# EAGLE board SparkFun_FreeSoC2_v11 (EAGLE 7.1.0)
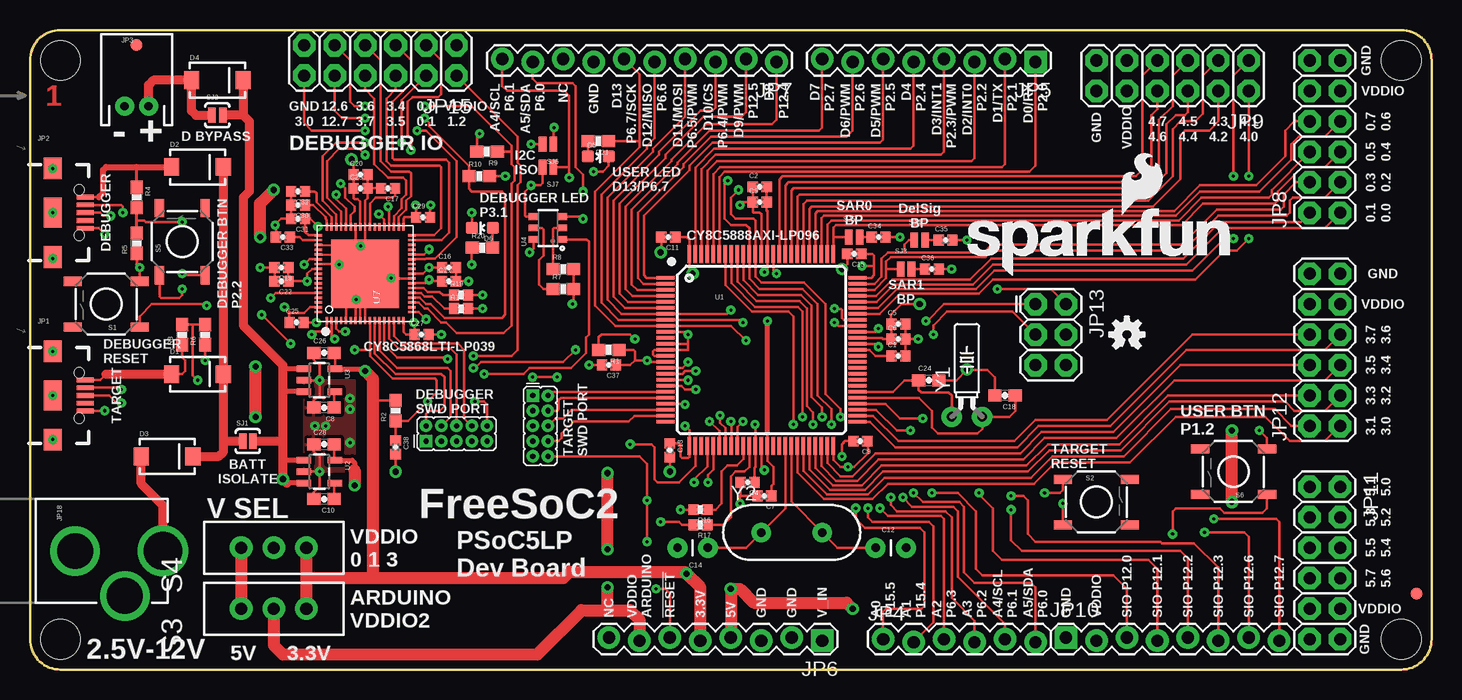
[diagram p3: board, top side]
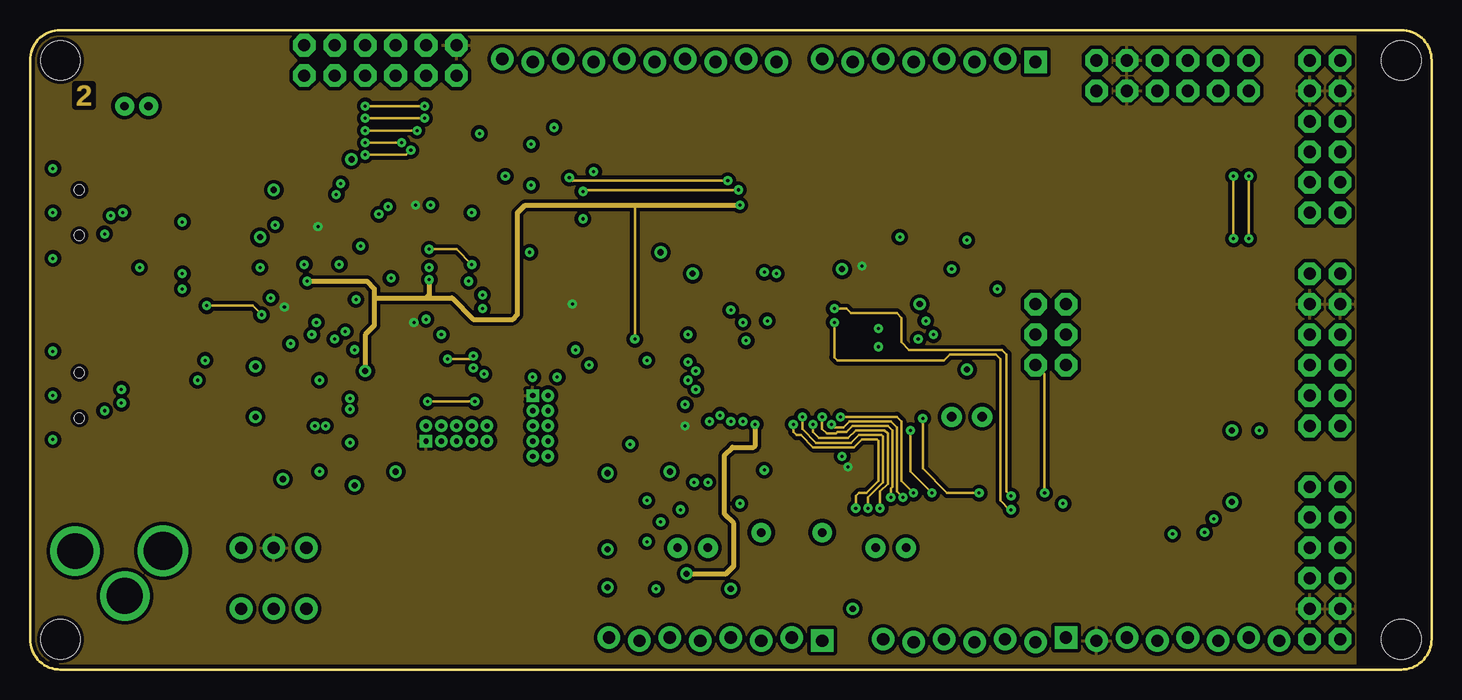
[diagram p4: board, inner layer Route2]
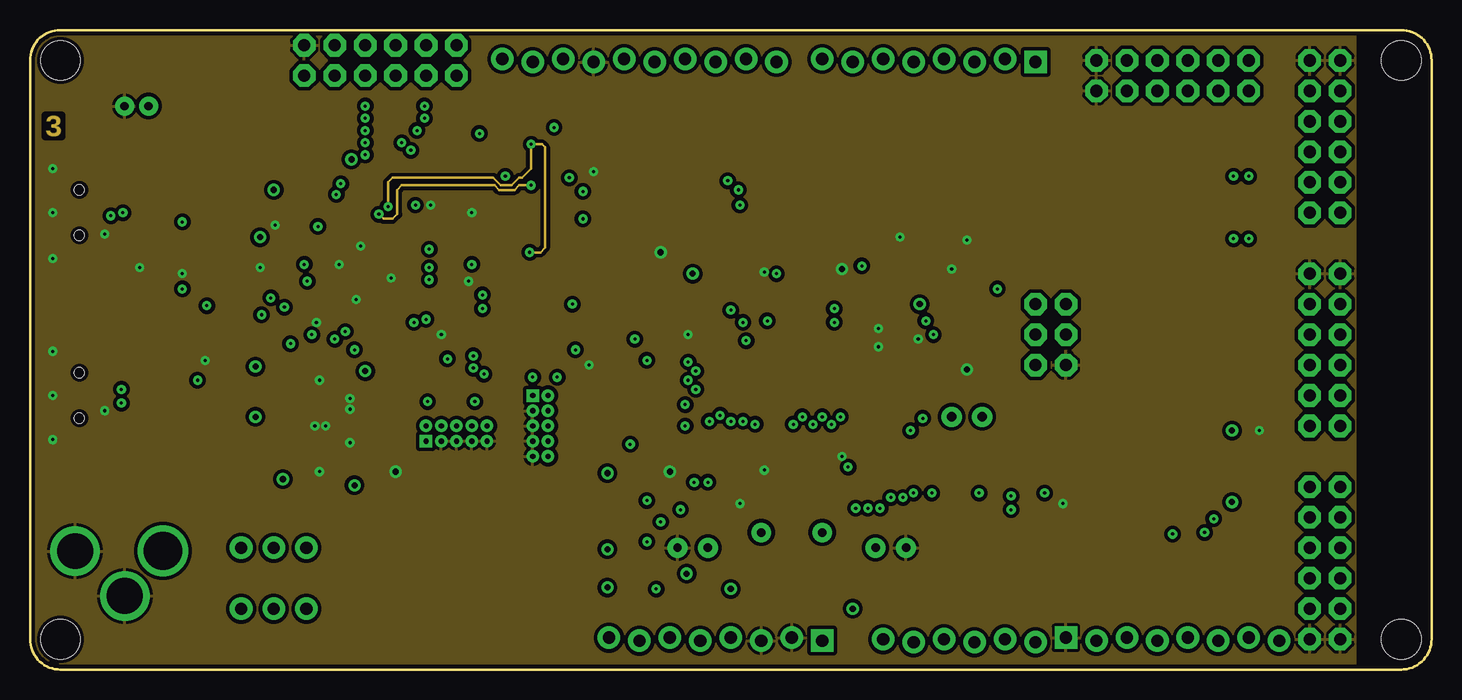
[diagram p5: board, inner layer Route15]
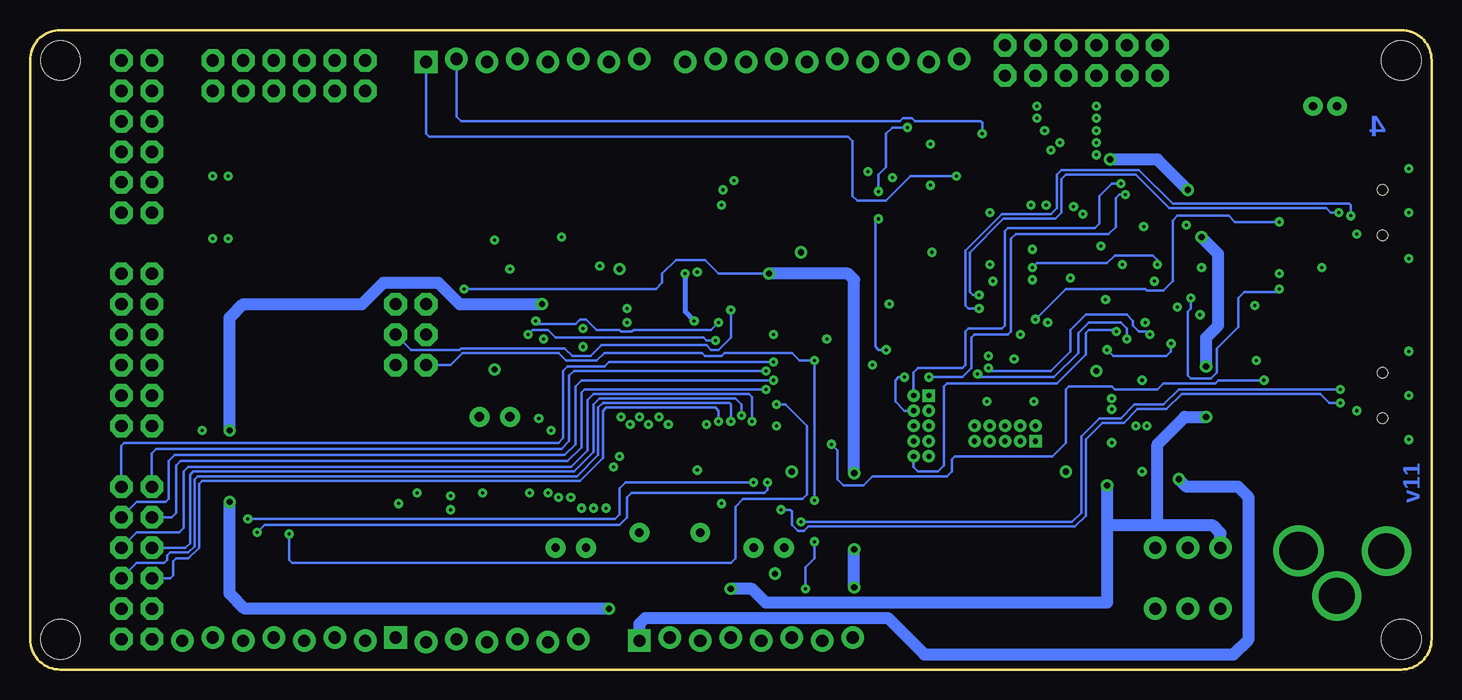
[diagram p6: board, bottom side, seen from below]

Size 116.84 x 53.34 mm. Coordinates in mm from the lower left corner, seen from the top.
Outline: 114.3,0 2.54,0 arc-90 0,2.54 0,50.8 arc-90 2.54,53.34 114.3,53.34 arc-90 116.84,50.8 116.84,2.54 arc-90 114.3,0
Copper layers (1*2*15*16): Top 0.035mm / dielectric 1.5mm / Route2 0.035mm / dielectric 0.15mm / Route15 0.035mm / dielectric 0.2mm / Bottom 0.035mm
Design rules "Sparkfun-x *": minimum track width 6mil, minimum drill 10mil, track to track 6mil, track to pad 6mil, pad to pad 6mil, via to via 8mil, smd to smd 6mil, copper to edge 6mil, drill to drill 8mil, minimum pad ring 12mil, minimum via ring 10mil, stop-mask expansion 4mil, vias tented up to drill 20mil, thermal gap 10mil
Net classes: 0 signal: width 0.203 mm, drill 0.254 mm, clearance 0.152 mm; 1 AVCC: width 0.508 mm, drill 0.508 mm, clearance 0.152 mm; 2 ARDUINO_VCC: width 0.508 mm, drill 0.381 mm

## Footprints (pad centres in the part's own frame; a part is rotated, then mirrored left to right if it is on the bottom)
0402-CAP = smd 0.85 x 0.9: 1 -0.58,0; 2 0.58,0
0603-CAP = smd 1.1 x 1: 1 -0.85,0; 2 0.85,0
CAP-PTH-SMALL = drill 0.7 pad 1.651: 1 0,0; 2 2.54,0
SMA-DIODE = smd 1.27 x 1.47: A -2.15,0; C 2.15,0
LED-0603 = smd 1 x 1: A 0,-0.877; C 0,0.877
FIDUCIAL-1X2 = smd 1 x 1: 1 0,0
USB-B-MICRO-SMD_V03 = smd 1.4 x 0.4: D+1 2.7,0; D-1 2.7,0.65; GND1 2.7,-1.3; ID1 2.7,-0.65; VBUS1 2.7,1.3 | smd 1.5 x 1.8: SHIELD1 0,3.7; SHIELD2 0,-3.7 | smd 1.5 x 2.5: SHIELD3 0,0 | hole 0.85: 2.2,1.9; 2.2,-1.9
JST-2-PTH = drill 0.7 pad 1.6: 1 -1,0; 2 1,0
1X06-SIP_LOCK = drill 1.016 pad 1.88: 1 0,0; 2 2.54,-0.254; 3 5.08,0; 4 7.62,-0.254; 5 10.16,0; 6 12.7,-0.254
1X08_LOCK = drill 1.016 pad 1.88 square: 1 0,0.127 | drill 1.016 pad 1.88: 2 2.54,-0.127; 3 5.08,0.127; 4 7.62,-0.127; 5 10.16,0.127; 6 12.7,-0.127; 7 15.24,0.127; 8 17.78,-0.127
1X10_LOCK = drill 1.016 pad 1.88: 1 0,0.127; 2 2.54,-0.127; 3 5.08,0.127; 4 7.62,-0.127; 5 10.16,0.127; 6 12.7,-0.127; 7 15.24,0.127; 8 17.78,-0.127; 9 20.32,0.127; 10 22.86,-0.127
2X6 = drill 1.016 pad 1.88 octagon: 1 0,0; 2 0,2.54; 3 2.54,0; 4 2.54,2.54; 5 5.08,0; 6 5.08,2.54; 7 7.62,0; 8 7.62,2.54; 9 10.16,0; 10 10.16,2.54; 11 12.7,0; 12 12.7,2.54
2X3 = drill 1.016 pad 1.88 octagon: 1 0,0; 2 0,2.54; 3 2.54,0; 4 2.54,2.54; 5 5.08,0; 6 5.08,2.54
2X5_PTH_SILK_.05 = drill 0.432 square: 1 0,6.35 | drill 0.432: 2 1.27,6.35; 3 0,5.08; 4 1.27,5.08; 5 0,3.81; 6 1.27,3.81; 7 0,2.54; 8 1.27,2.54; 9 0,1.27; 10 1.27,1.27
POWER_JACK_PTH_LOCK = drill 2.997 pad 4.115: GND 0.025,6.557; GNDBREAK 3.762,10.7 | drill 3.2 pad 4.115: PWR 0,13.878
0603-RES = smd 1.1 x 1: 1 -0.85,0; 2 0.85,0
0402-RES = smd 0.85 x 0.9: 1 -0.58,0; 2 0.58,0
TACTILE-SWITCH-SMD = smd 1.524 x 0.762: 1 -2.794,1.905; 2 2.794,1.905; 3 -2.794,-1.905; 4 2.794,-1.905
SWITCH-SPDT_LOCK.007S = drill 1.016 pad 1.88: 1 0,2.718; 2 0,0; 3 0,-2.718
PAD-JUMPER-2-NC_BY_PASTE_YES_SILK = smd 0.635 x 1.27: 1 -0.401,0; 2 0.413,0
PAD-JUMPER-2-NO_YES_SILK = smd 0.635 x 1.27: 1 -0.45,0; 2 0.45,0
PAD-JUMPER-2-NO_NO_SILK = smd 0.635 x 1.27: 1 -0.45,0; 2 0.45,0
STAND-OFF = hole 3.302: 0,0
TQFP-100-14X14MM = smd 1.5 x 0.27: 1 -8,6; 2 -8,5.5; 3 -8,5; 4 -8,4.5; 5 -8,4; 6 -8,3.5; 7 -8,3; 8 -8,2.5; 9 -8,2; 10 -8,1.5; 11 -8,1; 12 -8,0.5; 13 -8,0; 14 -8,-0.5; 15 -8,-1; 16 -8,-1.5; 17 -8,-2; 18 -8,-2.5; 19 -8,-3; 20 -8,-3.5; 21 -8,-4; 22 -8,-4.5; 23 -8,-5; 24 -8,-5.5; 25 -8,-6; 51 8,-6; 52 8,-5.5; 53 8,-5; 54 8,-4.5; 55 8,-4; 56 8,-3.5; 57 8,-3; 58 8,-2.5; 59 8,-2; 60 8,-1.5; 61 8,-1; 62 8,-0.5; 63 8,0; 64 8,0.5; 65 8,1; 66 8,1.5; 67 8,2; 68 8,2.5; 69 8,3; 70 8,3.5; 71 8,4; 72 8,4.5; 73 8,5; 74 8,5.5; 75 8,6 | smd 0.27 x 1.5: 26 -6,-8; 27 -5.5,-8; 28 -5,-8; 29 -4.5,-8; 30 -4,-8; 31 -3.5,-8; 32 -3,-8; 33 -2.5,-8; 34 -2,-8; 35 -1.5,-8; 36 -1,-8; 37 -0.5,-8; 38 0,-8; 39 0.5,-8; 40 1,-8; 41 1.5,-8; 42 2,-8; 43 2.5,-8; 44 3,-8; 45 3.5,-8; 46 4,-8; 47 4.5,-8; 48 5,-8; 49 5.5,-8; 50 6,-8; 76 6,8; 77 5.5,8; 78 5,8; 79 4.5,8; 80 4,8; 81 3.5,8; 82 3,8; 83 2.5,8; 84 2,8; 85 1.5,8; 86 1,8; 87 0.5,8; 88 0,8; 89 -0.5,8; 90 -1,8; 91 -1.5,8; 92 -2,8; 93 -2.5,8; 94 -3,8; 95 -3.5,8; 96 -4,8; 97 -4.5,8; 98 -5,8; 99 -5.5,8; 100 -6,8
SOT23-5 = smd 0.55 x 1.2: 1 -0.95,-1.3; 2 0,-1.3; 3 0.95,-1.3; 4 0.95,1.3; 5 -0.95,1.3
SOT26 = smd 0.55 x 0.8: D1 -0.95,1.2; D2 0.95,1.2; G1 -0.95,-1.2; G2 0.95,-1.2; S1 0,1.2; S2 0,-1.2
QFN-68 = smd 0.6 x 0.2: 1 -3.9,3.2; 2 -3.9,2.8; 3 -3.9,2.4; 4 -3.9,2; 5 -3.9,1.6; 6 -3.9,1.2; 7 -3.9,0.8; 8 -3.9,0.4; 9 -3.9,0; 10 -3.9,-0.4; 11 -3.9,-0.8; 12 -3.9,-1.2; 13 -3.9,-1.6; 14 -3.9,-2; 15 -3.9,-2.4; 16 -3.9,-2.8; 17 -3.9,-3.2; 35 3.9,-3.2; 36 3.9,-2.8; 37 3.9,-2.4; 38 3.9,-2; 39 3.9,-1.6; 40 3.9,-1.2; 41 3.9,-0.8; 42 3.9,-0.4; 43 3.9,0; 44 3.9,0.4; 45 3.9,0.8; 46 3.9,1.2; 47 3.9,1.6; 48 3.9,2; 49 3.9,2.4; 50 3.9,2.8; 51 3.9,3.2 | smd 0.2 x 0.6: 18 -3.2,-3.9; 19 -2.8,-3.9; 20 -2.4,-3.9; 21 -2,-3.9; 22 -1.6,-3.9; 23 -1.2,-3.9; 24 -0.8,-3.9; 25 -0.4,-3.9; 26 0,-3.9; 27 0.4,-3.9; 28 0.8,-3.9; 29 1.2,-3.9; 30 1.6,-3.9; 31 2,-3.9; 32 2.4,-3.9; 33 2.8,-3.9; 34 3.2,-3.9; 52 3.2,3.9; 53 2.8,3.9; 54 2.4,3.9; 55 2,3.9; 56 1.6,3.9; 57 1.2,3.9; 58 0.8,3.9; 59 0.4,3.9; 60 0,3.9; 61 -0.4,3.9; 62 -0.8,3.9; 63 -1.2,3.9; 64 -1.6,3.9; 65 -2,3.9; 66 -2.4,3.9; 67 -2.8,3.9; 68 -3.2,3.9 | smd 5.7 x 5.7: 69 0,0
TC26H = drill 0.813 pad 1.676: 1 -1.27,0; 2 1.27,0
HC49US = drill 0.7 pad 1.651: 1 -2.54,0; 2 2.54,0

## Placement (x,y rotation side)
C1  1.0uF  [0402-CAP]  72.39,26.16 0 top
C2  1.0uF  [0402-CAP]  60.83,40.26 0 top
C3  0.1uF  [0402-CAP]  60.83,38.99 0 top
C4  1.0uF  [0402-CAP]  59.82,15.62 180 top
C5  1.0uF  [0402-CAP]  72.39,28.83 0 top
C6  0.1uF  [0402-CAP]  72.39,27.56 0 top
C7  1.0uF  [0402-CAP]  61.21,14.48 180 top
C8  470pF  [0603-CAP]  24.51,21.84 180 top
C9  0.1uF  [0402-CAP]  69.22,19.05 180 top
C10  470pF  [0603-CAP]  24.51,14.22 180 top
C11  0.1uF  [0402-CAP]  53.21,36.07 180 top
C12  [CAP-PTH-SMALL]  70.48,10.16 0 top
C13  0.1uF  [0402-CAP]  53.34,18.29 270 top
C14  [CAP-PTH-SMALL]  56.52,10.16 180 top
C15  0.1uF  [0402-CAP]  68.71,34.67 180 top
C16  1.0uF  [0402-CAP]  34.92,33.53 0 top
C17  1.0uF  [0402-CAP]  29.84,40.13 180 top
C18  22pF  [0603-CAP]  81.28,22.86 180 top
C19  1.0uF  [0402-CAP]  20.95,33.53 180 top
C20  1.0uF  [0402-CAP]  27.56,41.27 0 top
C21  0.1uF  [0402-CAP]  34.92,32.38 0 top
C22  0.1uF  [0402-CAP]  20.95,32.38 180 top
C23  0.1uF  [0402-CAP]  27.56,40.13 0 top
C24  22pF  [0603-CAP]  74.93,24.13 0 top
C25  0.1uF  [0402-CAP]  22.23,28.96 0 top
C26  2.2uF  [0603-CAP]  24.51,26.42 0 top
C27  0.1uF  [0402-CAP]  32.64,27.94 0 top
C28  2.2uF  [0603-CAP]  24.51,18.8 0 top
C29  0.1uF  [0402-CAP]  32.77,37.72 0 top
C30  0.1uF  [0402-CAP]  22.35,38.73 180 top
C31  0.1uF  [0402-CAP]  22.35,37.59 180 top
C32  0.1uF  [0402-CAP]  22.35,39.88 180 top
C33  0.1uF  [0402-CAP]  21.08,36.07 180 top
C34  0.1uF  [0402-CAP]  70.74,36.07 0 top
C35  0.1uF  [0402-CAP]  76.33,35.81 0 top
C36  0.1uF  [0402-CAP]  75.18,33.4 0 top
C37  0.1uF  [0402-CAP]  48.26,25.4 180 top
C38  0.1uF  [0402-CAP]  30.48,18.54 270 top
D1  MBRA140  [SMA-DIODE]  13.97,24.64 0 top
D2  MBRA140  [SMA-DIODE]  13.97,41.91 0 top
D3  MBRA140  [SMA-DIODE]  11.43,17.78 0 top
D4  MBRA140  [SMA-DIODE]  15.62,49.15 0 top
D5  RED  [LED-0603]  47.37,42.8 270 top
D6  RED  [LED-0603]  37.72,36.83 90 top
FID1  FIDUCIAL1X2  [FIDUCIAL-1X2]  115.57,6.35 0 top
FID2  FIDUCIAL1X2  [FIDUCIAL-1X2]  8.89,52.07 0 top
FRAME1  [DUMMY]  not placed on the board
FRAME2  [DUMMY]  not placed on the board
FRAME3  [DUMMY]  not placed on the board
JP1  MicroB  [USB-B-MICRO-SMD_V03]  1.91,22.86 0 top
JP2  MicroB  [USB-B-MICRO-SMD_V03]  1.91,38.1 0 top
JP3  M02JST-PTH-2  [JST-2-PTH]  8.89,46.99 0 top
JP4  1X6 FEMALE PTH  [1X06-SIP_LOCK]  71.12,2.54 0 top
JP5  1X8 FEMALE PTH  [1X08_LOCK]  83.82,50.8 180 top
JP6  1X8 FEMALE PTH  [1X08_LOCK]  66.04,2.54 180 top
JP7  1X10 FEMALE PTH  [1X10_LOCK]  62.23,50.8 180 top
JP8  2X6 FEMALE  [2X6]  109.22,38.1 90 top
JP9  2X6 FEMALE  [2X6]  101.6,50.8 180 top
JP10  1x8 FEMALE PTH  [1X08_LOCK]  86.36,2.54 0 top
JP11  2X6 FEMALE  [2X6]  106.68,15.24 270 top
JP12  2X6 FEMALE  [2X6]  109.22,20.32 90 top
JP13  [2X3]  83.82,30.48 270 top
JP14  DNP  [2X5_PTH_SILK_.05]  39.37,19.05 90 top
JP15  2X6 FEMALE  [2X6]  35.56,52.07 180 top
JP17  DNP  [2X5_PTH_SILK_.05]  41.91,16.51 0 top
JP18  POWER_JACKPTH_LOCK  [POWER_JACK_PTH_LOCK]  -2.79,9.91 270 top
LOGO1  SFE_LOGO_NAME_FLAME.2_INCH  [SFE_LOGO_NAME_FLAME_.2]  77.47,32.77 0 top
LOGO2  OSHW-LOGOS  [OSHW-LOGO-S]  91.44,27.94 0 top
R1  4.7K  [0603-RES]  48.26,26.67 180 top
R2  4.7K  [0603-RES]  30.48,21.59 90 top
R3  10K  [0603-RES]  12.7,27.94 90 top
R4  10K  [0603-RES]  8.89,39.37 270 top
R5  20k  [0603-RES]  8.89,35.56 90 top
R6  20k  [0603-RES]  14.61,27.94 90 top
R7  2.2k  [0603-RES]  44.45,31.75 0 top
R8  2.2k  [0603-RES]  44.45,33.4 0 top
R9  1K  [0603-RES]  38.1,43.18 180 top
R10  1K  [0603-RES]  37.47,41.15 0 top
R16  22  [0402-RES]  55.88,13.34 180 top
R17  22  [0402-RES]  55.88,12.06 180 top
R18  22  [0402-RES]  35.94,30.1 0 top
R19  22  [0402-RES]  35.94,31.24 0 top
R20  1K  [0603-RES]  37.72,35.18 0 top
R21  1K  [0603-RES]  47.37,44.07 180 top
S1  SPST-MOM  [TACTILE-SWITCH-SMD]  6.35,30.48 180 top
S2  SPST-MOM  [TACTILE-SWITCH-SMD]  88.9,13.97 0 top
S3  SPDT  [SWITCH-SPDT_LOCK.007S]  20.32,5.08 90 top
S4  SPDT  [SWITCH-SPDT_LOCK.007S]  20.32,10.16 90 top
S5  SPST-MOM  [TACTILE-SWITCH-SMD]  12.7,35.69 90 top
S6  SPST-MOM  [TACTILE-SWITCH-SMD]  100.33,16.51 180 top
SJ1  JUMPER-PAD-2-NC_BY_PASTE  [PAD-JUMPER-2-NC_BY_PASTE_YES_SILK]  18.16,19.05 0 top
SJ2  JUMPER-PAD-2-NOYES_SILK  [PAD-JUMPER-2-NO_YES_SILK]  15.62,46.23 0 top
SJ3  JUMPER-PAD-2-NO  [PAD-JUMPER-2-NO_NO_SILK]  73.03,33.4 0 top
SJ4  JUMPER-PAD-2-NO  [PAD-JUMPER-2-NO_NO_SILK]  74.17,35.81 0 top
SJ5  JUMPER-PAD-2-NO  [PAD-JUMPER-2-NO_NO_SILK]  68.71,36.07 0 top
SJ6  JUMPER-PAD-2-NO  [PAD-JUMPER-2-NO_NO_SILK]  43.18,43.81 180 top
SJ7  JUMPER-PAD-2-NO  [PAD-JUMPER-2-NO_NO_SILK]  43.18,41.91 180 top
STANDOFF1  STAND-OFF  [STAND-OFF]  2.54,2.54 0 top
STANDOFF2  STAND-OFF  [STAND-OFF]  2.54,50.8 0 top
STANDOFF3  STAND-OFF  [STAND-OFF]  114.3,50.8 0 top
STANDOFF4  STAND-OFF  [STAND-OFF]  114.3,2.54 0 top
U1  CY8C5888AXI-LP096  [TQFP-100-14X14MM]  60.96,26.67 0 top
U2  MIC5219 5V  [SOT23-5]  24.13,16.51 270 top
U3  MIC5219 3.3V  [SOT23-5]  24.13,24.13 270 top
U4  2A/20V  [SOT26]  43.18,36.83 90 top
U7  CY8C5868LTI-LP039  [QFN-68]  27.94,33.02 90 top
U$1  FOUR_LAYER_WARNING  [FOUR_LAYER_WARNING]  15.24,-2.16 0 top
U$2  [CREATIVE_COMMONS]  not placed on the board
Y1  32.768kHz  [TC26H]  78.11,21.08 0 top
Y2  [HC49US]  63.5,11.43 0 top

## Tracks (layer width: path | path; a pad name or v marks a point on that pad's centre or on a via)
3.3V  (via drill 0.25, 0.51)
  Top 0.203: U3.5 25.43,26.35 C26.2 | R2.2 29,22.44 28.57,22.86 | C19.1 C22.1 v23.11,32.38 23.11,33.02 23.51,33.42 U7.59 | U7.24 32.98,32.22 v33.27,32.51 33.4,32.38 C21.1 | C4.1 60.4,16.84 60.47,16.91 U1.37 v60.46,20.44 v60.45,20.45 | U1.88 60.96,37.97 60.83,38.1 60.33,38.1 60.25,38.17 C3.1 | C2.1 C3.1 | C3.1 59.44,38.99 v59.18,38.73 | R1.2 47.41,27.73 47.62,27.94 50.04,27.94 v50.42,27.56
  Top 0.406: U3.5 27.75,25.08 v27.94,24.89
  Top 1.016: v27.94,24.89 28.57,24.26 28.57,22.86 28.57,7.75 28.45,7.62 | JP6.5 55.88,6.86 v54.74,8 54.61,8.13 44.96,8.13 44.45,7.62 28.45,7.62 | 28.45,7.62 23.04,7.62 | S4.3 23.04,7.62 | 23.04,7.62 S3.3
  Route2 0.203: v50.42,27.56 50.42,38.73
  Route2 0.406: v23.11,32.38 28.07,32.38 28.7,31.75 28.7,30.99 | 28.7,30.99 28.7,28.7 27.94,27.94 v27.94,24.89 | v54.74,8 58.04,8 58.67,8.64 58.67,12.19 57.91,12.95 57.91,17.91 58.55,18.54 60.33,18.54 U1.37 v60.46,20.44 v60.45,20.45 | 57.78,38.73 v59.18,38.73 50.42,38.73 41.27,38.73 40.64,38.1 40.64,29.59 40.26,29.21 36.96,29.21 35.18,30.99 33.02,30.99 | 28.7,30.99 33.02,30.99 | v33.27,32.51 33.27,31.24 33.02,30.99
5V  (via drill 0.51)
  Top 0.203: C28.2 25.36,17.53 U2.5 | U1.65 71.01,27.67 71.12,27.56 C6.1 C5.1 71.81,29.16 71.75,29.21 | 71.75,29.21 71.75,29.59 72.64,30.48 v74.17,30.48 | 71.75,29.21 71.75,28.84 | U7.44 27.54,39.01 27.3,39.24 27.05,39.24 26.98,39.31 C23.1 C20.1 26.98,42.36 v26.8,42.55 26.91,42.43
  Top 0.406: U2.5 26.86,17.46 27.05,17.27 27.05,16.64
  Top 1.016: S4.1 S3.1 | 27.05,16.64 v27.05,15.37 | JP6.4 v58.42,6.73 59.18,6.73 60.33,5.59 68.07,5.59 v68.58,5.08 | v100.2,13.97 v100.2,19.94 | v18.8,21.08 v18.8,25.27 | v19.18,36.07 19.18,38.86 v20.32,40.01
  Bottom 1.016: 27.05,12.06 22.86,12.06 | 22.86,12.06 18.29,12.06 17.6,11.38 S4.1 | v27.05,15.37 27.05,12.06 | 27.05,12.06 27.05,5.59 55.5,5.59 56.64,6.73 v58.42,6.73 | v68.58,5.08 98.93,5.08 100.2,6.35 v100.2,13.97 | v100.2,19.94 100.2,29.34 99.06,30.48 89.15,30.48 87.38,32.26 82.8,32.26 81.03,30.48 v74.17,30.48 | 22.86,12.06 22.86,18.8 20.57,21.08 v18.8,21.08 | v18.8,25.27 18.8,27.69 17.78,28.7 17.78,34.67 v19.18,36.07 | v20.32,40.01 22.86,42.55 v26.8,42.55
!DEBUG_P2.6_SCL_PU_EN  (via drill 0.25)
  Top 0.203: U7.1 24.74,28.55 24.38,28.19 23.75,28.19 v23.5,27.94 | v36.96,25.15 37.08,25.15 37.59,25.65 44.45,25.65 v45.47,26.67 | U4.G2 45.91,37.78 v46.1,37.59
  Bottom 0.203: v23.5,27.94 23.75,28.19 24.38,28.19 24.89,28.7 24.89,29.08 25.4,29.59 28.83,29.59 30.1,28.32 30.1,26.54 31.75,24.89 36.7,24.89 v36.96,25.15 | v45.47,26.67 46.1,26.67 46.35,26.92 46.35,37.34 v46.1,37.59
!DEBUG_P2.7_SDA_PU_EN  (via drill 0.25)
  Top 0.203: U7.2 25.14,27.82 v25.4,27.56 | v37.85,24.64 41.15,24.64 41.66,25.15 45.09,25.15 46.35,26.42 46.35,27.69 46.61,27.94 46.61,35.69 46.42,35.88 U4.G1
  Bottom 0.203: v25.4,27.56 25.4,28.45 25.91,28.96 28.57,28.96 29.46,28.07 29.46,26.42 31.5,24.38 37.59,24.38 v37.85,24.64
!DEBUG_RESET  (via drill 0.25)
  Top 0.203: U7.10 28.34,26.67 | 28.34,26.67 28.34,26.14 30.23,24.26 33.78,24.26 33.91,24.13 33.91,23.11 v33.15,22.35 31.54,20.74 R2.1 C38.1 | v37.08,22.35 37.85,22.35 38.1,22.1 JP14.10 | S1.1 9.14,29.46 10.16,30.48 14.61,30.48 v14.73,30.35 | v19.3,29.59 v21.72,27.18 | v27.05,26.67 28.34,26.67
  Route2 0.203: v33.15,22.35 v37.08,22.35 | v14.73,30.35 18.54,30.35 v19.3,29.59
  Bottom 0.203: v21.72,27.18 21.72,26.54 22.1,26.16 26.54,26.16 v27.05,26.67
!RESET  (via drill 0.25)
  Top 0.203: U1.15 51.55,25.67 v51.44,25.78 50.42,25.78 | v84.58,14.73 85.85,14.73 86.11,14.99 S2.1 | v51.44,10.67 v51.44,14.1 51.44,17.14 50.8,17.78 JP17.10 | v52.2,6.73 52.96,6.73 53.34,6.35 JP6.6 | U7.3 25.54,28.43 25.78,28.19 v26.29,28.19 | C37.1 50.04,25.4 50.42,25.78 | R1.1 50.29,26.67 50.42,26.54 50.42,25.78
  Route2 0.203: JP13.5 84.58,24.64 v84.58,14.73
  Bottom 0.203: v51.44,14.1 v51.44,25.78 52.7,25.78 53.34,26.42 58.93,26.42 59.18,26.16 60.58,26.16 60.83,26.42 68.96,26.42 69.6,25.78 72.14,25.78 72.77,26.42 80.77,26.42 81.79,25.4 JP13.5 | JP17.10 43.18,16.89 42.8,16.51 41.15,16.51 40.64,17.02 40.64,23.62 40.39,23.88 31.24,23.88 28.83,26.29 28.83,28.07 28.57,28.32 26.42,28.32 v26.29,28.19 | v51.44,10.67 51.44,9.27 52.2,8.51 v52.2,6.73
A0  (via drill 0.25)
  Top 0.203: U1.94 57.96,32.08 60.2,29.84 63.25,29.84 63.63,29.46 v63.63,20.45 | v68.83,13.46 68.83,12.57 69.6,11.81 74.17,11.81 74.55,11.43 74.55,5.33 74.3,5.08 71.37,5.08 71.12,4.83 JP4.1
  Route2 0.203: v63.63,20.45 63.63,19.81 63.88,19.56 64.26,19.56 65.28,18.54 68.71,18.54 69.34,19.18 70.61,19.18 70.74,19.05 70.74,15.75 69.72,14.73 69.09,14.73 68.83,14.48 v68.83,13.46
A1  (via drill 0.25)
  Top 0.203: U1.93 58.46,32.22 60.45,30.23 64.01,30.23 64.39,29.84 v64.39,21.08 | v69.85,13.46 69.85,12.7 70.23,12.32 74.93,12.32 75.31,11.94 75.31,3.94 JP4.2
  Route2 0.203: v64.39,21.08 64.39,20.07 65.53,18.92 68.45,18.92 69.09,19.56 70.99,19.56 71.12,19.43 71.12,15.62 69.85,14.35 v69.85,13.46
A2  (via drill 0.25)
  Top 0.203: U1.92 58.96,32.35 60.58,30.73 64.14,30.73 64.77,30.1 64.77,21.97 65.28,21.46 v65.28,20.45 | v70.87,13.46 71.5,12.83 75.95,12.83 76.2,12.57 JP4.3
  Route2 0.203: v65.28,20.45 65.28,19.81 65.79,19.3 68.2,19.3 68.83,19.94 71.25,19.94 71.5,19.68 71.5,15.49 70.87,14.86 v70.87,13.46
A3  (via drill 0.25)
  Top 0.203: U1.91 59.46,32.49 60.71,31.24 64.26,31.24 65.15,30.35 65.15,22.73 66.04,21.84 v66.04,21.08 | v71.75,14.35 71.75,13.72 72.26,13.21 76.33,13.21 76.83,12.7 76.83,5.97 78.74,4.06 JP4.4
  Route2 0.203: v66.04,21.08 66.04,20.07 66.42,19.68 67.18,19.68 67.31,19.81 68.07,19.81 68.58,20.32 71.5,20.32 71.88,19.94 71.88,15.24 71.75,15.11 v71.75,14.35
A4  (via drill 0.25)
  Top 0.203: v66.8,20.45 66.8,21.72 65.66,22.86 65.66,30.48 64.39,31.75 60.83,31.75 59.96,32.62 U1.90 59.96,36.81 59.69,37.08 58.42,37.08 57.91,37.59 57.91,40.51 v58.17,40.77 | v72.77,14.35 73.53,13.59 76.96,13.59 77.34,13.21 77.34,7.75 81.28,3.81 JP4.5 | v44.96,41.02 44.96,41.91 | 44.96,41.91 44.96,47.88 44.58,48.26 39.75,48.26 39.37,48.64 JP7.10 | SJ7.1 44.96,41.91
  Route2 0.203: v66.8,20.45 67.06,20.19 67.82,20.19 68.33,20.7 71.75,20.7 72.26,20.19 72.26,14.86 v72.77,14.35 | v58.17,40.77 45.21,40.77 v44.96,41.02
A5  (via drill 0.25)
  Top 0.203: v59.05,40.01 58.42,39.37 58.42,37.97 58.8,37.59 60.33,37.59 60.46,37.46 U1.89 60.46,32.76 60.96,32.26 64.52,32.26 66.29,30.48 66.29,22.99 67.56,21.72 v67.56,21.08 | v46.1,39.88 46.1,41.27 45.47,41.91 45.47,48.64 45.21,48.9 42.29,48.9 41.91,49.28 JP7.9 | v73.66,14.73 74.42,13.97 77.47,13.97 77.85,13.59 77.85,8.13 78.74,7.24 83.44,7.24 83.82,6.86 JP4.6 | SJ6.1 43.63,45.15 v43.69,45.21
  Route2 0.203: v67.56,21.08 72.26,21.08 72.64,20.7 72.64,15.75 v73.66,14.73 | v59.05,40.01 46.23,40.01 v46.1,39.88
  Bottom 0.203: v43.69,45.21 44.96,45.21 45.47,44.7 45.47,41.91 46.1,41.27 v46.1,39.88
D0  (via drill 0.25)
  Top 0.203: U1.95 57.46,41.08 57.91,41.53 83.31,41.53 83.82,42.04 JP5.1 | R10.2 v39.62,41.15
  Bottom 0.203: JP5.1 83.82,44.7 83.57,44.45 48.64,44.45 48.26,44.07 48.26,39.5 47.88,39.12 45.47,39.12 43.43,41.15 v39.62,41.15
D1  (via drill 0.25)
  Top 0.203: U1.96 56.96,41.34 57.53,41.91 81.03,41.91 81.28,42.16 JP5.2 | R9.2 37.25,44.49 v37.47,44.7
  Bottom 0.203: v37.47,44.7 37.47,45.59 37.59,45.72 43.05,45.72 43.31,45.97 44.07,45.97 44.32,45.72 80.9,45.72 81.28,46.1 JP5.2
D2
  Top 0.203: U1.97 56.46,41.6 57.28,42.42 78.49,42.42 78.74,42.67 JP5.3
D3
  Top 0.203: U1.98 55.96,41.74 57.15,42.93 75.95,42.93 76.2,43.18 JP5.4
D4
  Top 0.203: U1.99 55.46,41.87 57.02,43.43 73.41,43.43 73.66,43.69 JP5.5
D5
  Top 0.203: U1.1 51.4,32.67 51.18,32.89 51.18,37.85 54.99,41.66 54.99,42.04 56.9,43.94 70.87,43.94 71.12,44.2 JP5.6
D6
  Top 0.203: U1.2 51.14,32.17 50.67,32.64 50.67,38.1 54.48,41.91 54.48,42.16 56.77,44.45 68.07,44.45 68.58,44.96 JP5.7
D7
  Top 0.203: JP5.8 66.04,45.21 65.79,44.96 56.64,44.96 53.98,42.29 53.98,42.16 50.16,38.35 50.16,32.13 50.63,31.67 U1.3
D8
  Top 0.203: U1.4 50.24,31.17 49.66,31.75 49.66,38.61 53.47,42.42 53.47,42.55 56.39,45.47 61.85,45.47 62.23,45.85 JP7.1
D9
  Top 0.203: JP7.2 59.69,46.48 59.31,46.1 56.13,46.1 52.96,42.93 52.96,42.67 49.15,38.86 49.15,31.37 49.85,30.67 U1.5
D10
  Top 0.203: U1.6 49.59,30.17 48.64,31.11 48.64,39.12 52.45,42.93 52.45,43.18 55.88,46.61 56.9,46.61 57.15,46.86 JP7.3
D11  (via drill 0.25)
  Top 0.203: JP7.4 54.61,46.1 51.94,43.43 51.94,43.18 48.13,39.37 48.13,30.86 49.32,29.67 U1.7 58.12,29.67 v58.42,29.97
  Bottom 0.203: v58.42,29.97 58.42,27.69 59.44,26.67 60.07,26.67 60.45,27.05 69.22,27.05 70.1,26.16 71.63,26.16 72.26,26.8 80.9,26.8 81.03,26.67 85.09,26.67 JP13.4
D12  (via drill 0.25)
  Top 0.203: JP7.5 52.07,44.32 51.44,43.69 51.44,43.43 47.62,39.62 47.62,30.61 49.06,29.17 U1.8 59.22,29.17 v59.44,28.96 | v74.68,29.08 74.8,29.08 76.2,30.48 JP13.1
  Bottom 0.203: v59.44,28.96 60.07,28.32 66.55,28.32 66.67,28.19 67.56,28.19 67.69,28.32 69.6,28.32 70.48,29.21 70.99,29.21 71.37,28.83 74.42,28.83 v74.68,29.08
D13  (via drill 0.25)
  Top 0.203: 50.8,44.07 50.8,43.56 47.12,39.88 47.12,30.35 48.8,28.67 U1.9 58.45,28.67 v59.69,27.43 | 50.8,44.07 50.8,49.66 JP7.6 | R21.1 50.8,44.07 | v75.31,27.94 75.31,28.7 76.45,29.84 81.92,29.84 JP13.3
  Bottom 0.203: v59.69,27.43 60.45,27.43 60.71,27.69 73.03,27.69 73.66,28.32 74.93,28.32 v75.31,27.94
DEBUG_BTN  (via drill 0.25)
  Top 0.203: U7.64 20.5,31.42 v20.07,30.99 | v12.7,31.75 12.7,31.24 12.45,30.99 10.92,30.99 10.79,31.11 S5.1
  Bottom 0.203: v20.07,30.99 20.07,30.1 20.32,29.84 20.32,24.51 20.07,24.26 18.41,24.26 17.91,24.77 17.91,26.8 16.13,28.57 16.13,30.99 15.62,31.5 12.95,31.5 v12.7,31.75
DEBUG_D+_BUS  (via drill 0.25)
  Top 0.203: JP2.D+1 5.84,38.1 6.1,37.85 v6.73,37.85 | 37.47,30.1 v37.72,30.1 R18.2
  Bottom 0.203: v6.73,37.85 6.73,38.73 6.86,38.86 21.59,38.86 24.38,41.66 30.86,41.66 31.24,41.27 31.24,38.48 31.75,37.97 35.81,37.97 38.86,34.92 38.86,30.35 38.61,30.1 v37.72,30.1
DEBUG_D+_PAD
  Top 0.203: U7.22 32.59,31.42 32.89,31.11 33.53,31.11 34.54,30.1 R18.1
DEBUG_D-_BUS  (via drill 0.25)
  Top 0.203: JP2.D-1 7.61,38.75 7.75,38.61 v7.75,38.1 | v37.72,31.24 R19.2
  Bottom 0.203: v7.75,38.1 8.38,38.1 8.76,38.48 21.84,38.48 24.64,41.27 30.48,41.27 30.86,40.89 30.86,38.1 31.37,37.59 35.69,37.59 38.48,34.8 38.48,31.5 38.23,31.24 v37.72,31.24
DEBUG_D-_PAD
  Top 0.203: U7.23 32.82,31.82 33.15,31.5 34.16,31.5 34.42,31.24 R19.1
DEBUG_DS_BP
  Top 0.203: U7.51 24.74,37.49 24.64,37.59 24.64,37.72 23.62,38.73 C30.1
DEBUG_LED  (via drill 0.25)
  Top 0.203: U7.30 32.84,34.62 v33.27,35.05 | v36.83,33.78 36.83,35.14 R20.1
  Route2 0.203: v33.27,35.05 35.56,35.05 v36.83,33.78
DEBUG_P0.0  (via drill 0.25)
  Top 0.203: U7.48 25.94,38.2 24.77,39.37 24.77,42.42 25.78,43.43 27.43,43.43 v27.94,42.93 | v31.75,43.31 31.75,44.32 31.5,44.58 31.5,47.37 31.88,47.75 34.04,47.75 34.29,48.01 34.29,50.8 JP15.3
  Route2 0.203: v27.94,42.93 31.37,42.93 v31.75,43.31
DEBUG_P0.1  (via drill 0.25)
  Top 0.203: U7.49 25.54,37.96 24.38,39.12 24.38,42.8 25.53,43.94 v27.94,43.94 | v30.99,43.94 30.99,47.5 JP15.4
  Route2 0.203: v27.94,43.94 v30.99,43.94
DEBUG_P1.2  (via drill 0.25)
  Top 0.203: U7.13 29.54,27.1 30.61,26.04 34.67,26.04 v34.8,25.91 | v36.96,26.16 40.13,26.16 40.64,26.67 40.64,40.39 40.89,40.64 40.89,42.04 40.64,42.29 40.64,44.45 JP15.2
  Route2 0.203: v34.8,25.91 36.7,25.91 v36.96,26.16
DEBUG_P3.0  (via drill 0.25)
  Top 0.203: U7.29 32.95,34.22 33.02,34.29 33.78,34.29 35.56,36.07 35.56,42.42 33.02,44.96 v32.26,44.96 | v27.94,44.96 23.5,44.96 22.86,45.59 JP15.12
  Route2 0.203: v32.26,44.96 v27.94,44.96
DEBUG_P3.4
  Top 0.203: U7.33 34.3,35.82 34.92,36.45 34.92,42.29 34.67,42.55 30.35,42.55 30.23,42.67 30.23,47.37 31.75,48.9 31.75,50.8 JP15.5
DEBUG_P3.5
  Top 0.203: U7.34 33.68,36.22 34.29,36.83 34.29,41.91 34.16,42.04 30.1,42.04 29.72,42.42 29.72,47.62 30.48,48.39 JP15.6
DEBUG_P3.6
  Top 0.203: JP15.7 29.21,50.8 29.21,42.42 30.1,41.53 31.62,41.53 31.75,41.4 31.75,39.5 31.37,39.12 31.37,38.35 30.74,37.73 U7.36
DEBUG_P3.7
  Top 0.203: JP15.8 27.94,48.39 28.7,47.62 28.7,42.16 29.84,41.02 31.11,41.02 31.37,40.77 31.37,39.62 30.99,39.24 30.99,38.48 30.34,37.83 U7.37
DEBUG_P12.0_SCL  (via drill 0.25)
  Top 0.203: U7.39 29.54,37.52 v29.08,37.97 | U4.D2 41.34,37.78 41.27,37.85 41.27,39.88 v41.78,40.39 42.55,40.39 42.73,40.57 SJ7.2
  Route15 0.203: v41.78,40.39 40.77,40.39 40.39,40.01 39.12,40.01 38.73,40.39 30.99,40.39 30.61,40.01 30.61,37.97 30.23,37.59 29.46,37.59 v29.08,37.97
DEBUG_P12.1_SDA  (via drill 0.25)
  Top 0.203: U7.38 29.94,38.51 v29.84,38.61 | U4.D1 41.98,35.12 v41.66,34.8 | v41.78,43.81 SJ6.2
  Route15 0.203: v41.66,34.8 42.55,34.8 42.93,35.18 42.93,43.56 42.67,43.81 v41.78,43.81 41.78,41.78 41.02,41.02 40.77,41.02 40.13,40.39 39.24,40.39 38.61,41.02 30.23,41.02 29.84,40.64 v29.84,38.61
DEBUG_P12.6_RX  (via drill 0.25)
  Top 0.203: 40.13,43.18 40.13,42.16 40.39,41.91 40.39,40.77 40.13,40.51 40.13,28.7 39.5,28.07 35.56,28.07 34.67,28.96 34.29,28.96 33.15,30.1 32.89,30.1 32.38,30.61 31.85,30.61 U7.20 | 40.13,43.18 40.13,43.69 36.83,46.99 v32.89,46.99 | v27.94,46.99 27.05,46.99 26.67,47.37 26.67,50.8 JP15.9 | R9.1 40.13,43.18
  Route2 0.203: v32.89,46.99 v27.94,46.99
DEBUG_P12.7_TX  (via drill 0.25)
  Top 0.203: v27.94,45.97 26.04,45.97 25.4,46.61 JP15.10 | U7.21 32.48,31.02 33.02,30.48 33.4,30.48 34.54,29.34 39.37,29.34 39.62,29.59 39.62,39.62 39.37,39.88 36.83,39.88 36.62,40.09 R10.1 36.62,42 33.27,45.34 33.27,45.59 v32.89,45.97
  Route2 0.203: v32.89,45.97 v27.94,45.97
DEBUG_SAR0_BP
  Top 0.203: U7.53 22.73,35.82 22.48,36.07 C33.1
DEBUG_SAR1_BP
  Top 0.203: C32.1 23.75,39.88 23.88,39.75 23.88,38.99 25.15,37.72 25.14,37.71 U7.50
DEBUG_SWDCK_TCK
  Top 0.203: U7.12 29.14,26.61 30.61,25.15 34.8,25.15 35.05,24.89 35.05,21.08 JP14.4
DEBUG_SWDIO_TMS
  Top 0.203: U7.11 28.74,26.38 30.48,24.64 34.29,24.64 34.54,24.38 34.54,21.97 34.16,21.59 33.27,21.59 33.02,21.34 JP14.2
DEBUG_SWV_TDO
  Top 0.203: JP14.6 35.56,26.29 35.05,26.8 30.73,26.8 29.94,27.59 U7.14
DEBUG_TDI
  Top 0.203: U7.15 30.34,27.83 30.99,27.18 35.69,27.18 36.2,26.67 36.2,20.95 JP14.8
GND  (via drill 0.25, 0.51)
  Top 0.152: 26.67,35.56 25.4,35.56 25.26,35.42 U7.54 27,35.42 27.14,35.56 | U7.56 26.81,34.62 27.14,34.29
  Top 0.203: C2.2 C3.2 61.41,38.27 61.46,38.22 U1.87 61.46,33.39 v61.21,33.15 | S2.3 v86.11,13.84 | U1.66 70.46,28.17 v70.74,28.45 | U1.10 54.63,28.17 v54.86,27.94 54.86,27.18 54.86,27.17 | U1.12 54.86,27.17 | 54.86,27.17 54.86,27.16 54.86,26.67 U1.13 52.07,26.67 51.94,26.54 51.94,26.29 52.06,26.17 U1.14 | JP1.GND1 6.19,21.56 v6.22,21.59 | JP2.GND1 5.75,36.8 v6.22,36.32 | S1.3 v9.14,33.53 | U7.25 28.34,32.62 U7.69 | U7.9 U7.69 | U7.58 27.14,33.82 | U7.45 27.14,35.56 27.14,34.29 27.14,33.82 | 27.14,33.82 U7.69 | U7.7 27.14,32.22 U7.69 | U7.5 26.34,32.69 26.67,33.02 U7.69 | U7.8 27.54,32.62 U7.69 | U3.2 v24.13,24.13 | v24.13,24.13 24.13,25.4 23.66,25.87 C26.1 | C8.2 23.66,22.39 24.13,22.86 v24.13,24.13 | U2.2 v24.13,16.51 | v24.13,16.51 24.13,17.78 23.66,18.25 C28.1 | C10.2 23.66,14.77 24.13,15.24 v24.13,16.51 | v25.78,33.78 27.18,33.78 U7.69 | v67.69,33.4 68.13,33.84 C15.2 | v1.91,19.18 JP1.SHIELD2 | v1.91,26.54 JP1.SHIELD1 | v1.91,34.29 JP2.SHIELD2 | JP2.SHIELD1 v1.91,41.78 | U7.69 U7.43 27.93,36.94 27.93,39.1 28.14,39.31 C23.2 | U1.64 70.49,27.17 v70.74,26.92 | C5.2 C6.2 | C1.2 C6.2 | v74.04,27.56 C6.2 | U1.38 60.96,16.89 v61.21,16.64 | 52.56,34.81 v52.58,34.8 52.63,34.85 C11.2 | C9.2 67.94,19.05 67.69,18.8 v67.69,17.78 | 20.43,37.07 v20.45,37.08 | v20.45,37.08 20.95,37.59 C31.2 C30.2 C32.2 | D6.C 36.84,38.09 v36.83,38.1 | C36.2 v76.83,33.4 | C34.2 v72.52,36.07 | C35.2 v78.11,35.81 | 59.17,14.48 59.17,13.86 v59.18,13.84 | C7.2 59.17,14.48 | D5.C 48.25,42.02 47.75,41.53 v46.99,41.53 | S6.3 103.12,19.3 v102.49,19.94 | 33.42,38.72 v33.4,38.73 33.35,38.68 C29.2 | C16.2 C21.2 v36.58,32.38 | C27.2 v34.29,27.94 | C25.2 v23.88,28.96 | C22.2 C19.2 20.36,33.54 19.19,33.54 v19.18,33.53
  Top 0.203: S5.3 12.83,32.89 v12.7,33.02 | C20.2 C23.2 | C18.2 80.43,24.34 79.8,24.98 78.14,24.98 v78.11,25.02 77.22,24.13 C24.2 | C38.2 v30.48,16.51 | R6.1 v14.61,25.78 | C13.2 v53.34,16.51 | C33.2 20.5,37.03 v20.45,37.08 | C4.2 59.24,14.55 59.17,14.48 | C23.2 C17.2 | C37.2 v46.61,25.4
  Top 0.254: R5.1 8.89,33.78 v9.14,33.53
  other vias: 1.91,22.86 1.91,38.1 27.18,30.86 27.56,35.31 30.1,32.64 26.67,21.72 26.67,22.61 26.67,18.92 24.64,20.32 23.75,20.32
  pour Route15 (isolate 0.305): 0,53.34 110.49,53.34 110.49,0 0,0
  pour Top (isolate 0.305): 27.05,24.13 27.05,16.51 22.86,16.51 22.86,24.13
N$1
  Top 0.203: C8.1 25.36,23.11 U3.4
N$2
  Top 0.203: C10.1 25.36,15.49 U2.4
N$3
  Top 0.203: SJ5.2 C34.1
N$4
  Top 0.203: SJ4.2 C35.1
N$5
  Top 0.203: SJ3.2 C36.1
N$7
  Top 0.203: R8.1 43.6,36.74 43.69,36.83 U4.S2
N$8
  Top 0.203: U4.S1 42.67,36.83 42.8,36.7 42.8,34.54 42.42,34.16 42.42,32.13 42.8,31.75 R7.1
N$13
  Top 0.762: D3.A 9.27,15.49 10.48,14.29 10.91,13.86 11.08,13.68 JP18.PWR
N$14  (via drill 0.25)
  Top 0.203: U7.26 32.77,33.02 v33.27,33.53 C16.1 | U7.57 23.3,34.22 v22.86,33.78
  Bottom 0.203: v33.27,33.53 32.89,33.91 27.05,33.91 26.42,34.54 23.24,34.54 22.86,34.16 v22.86,33.78
N$16
  Top 0.406: 17.53,19.05 SJ1.1
  Top 0.762: D2.C D1.C 16.12,24.26 | 16.12,24.26 16.12,23.74 | D3.C 15.75,17.78 16.13,18.16 16.13,18.92 | 16.13,18.92 16.13,24.25 16.12,24.26 | 16.13,18.92 16.26,19.05 17.53,19.05
N$17
  Top 0.406: 14.99,46.23 SJ2.1
  Top 0.762: JP3.2 9.89,48.75 10.29,49.15 D4.A 13.46,46.61 13.84,46.23 14.99,46.23
N$23
  Top 0.203: R20.2 38.57,36.8 D6.A
N$26
  Top 0.203: R21.2 46.52,42.83 D5.A
N$27
  Top 0.203: U7.42 28.34,38.88 28.83,39.37 30.23,39.37 30.43,39.57 C17.1
P0.0
  Top 0.203: U1.71 70.55,30.67 72.01,32.13 78.61,32.13 80.26,33.78 96.39,33.78 99.44,36.83 107.95,36.83 JP8.1
P0.1
  Top 0.203: U1.72 70.54,31.17 71.88,32.51 78.36,32.51 80.14,34.29 96.14,34.29 99.19,37.34 105.92,37.34 JP8.2
P0.2
  Top 0.203: U1.73 70.41,31.67 71.37,32.64 71.37,33.4 | 71.37,33.4 71.37,34.04 71.75,34.42 79.63,34.42 80.14,34.92 96.14,34.92 99.06,37.85 104.78,37.85 105.03,38.1 105.03,39.12 105.28,39.37 107.95,39.37 JP8.3 | SJ3.1 71.37,33.4
P0.3
  Top 0.203: U1.74 70.4,32.17 70.99,32.77 70.99,34.29 71.5,34.8 72.9,34.8 | 72.9,34.8 79.5,34.8 80.14,35.43 96.01,35.43 98.93,38.35 104.27,38.35 104.52,38.61 104.52,39.62 105.54,40.64 JP8.4 | SJ4.1 73.28,35.81 72.9,35.43 72.9,34.8
P0.4
  Top 0.203: U1.76 66.96,36.07 | 66.96,36.07 66.96,36.86 67.18,37.08 96.01,37.08 97.79,38.86 103.76,38.86 104.01,39.12 104.01,39.88 106.05,41.91 107.95,41.91 JP8.5 | SJ5.1 66.96,36.07
P0.5
  Top 0.203: U1.77 66.46,37.12 66.8,37.47 95.76,37.47 97.66,39.37 103.25,39.37 103.5,39.62 103.5,40.01 JP8.6
P0.6
  Top 0.203: U1.78 65.96,37.64 66.17,37.85 95.5,37.85 97.54,39.88 102.49,39.88 105.16,42.55 105.16,43.81 105.79,44.45 107.95,44.45 JP8.7
P0.7
  Top 0.203: U1.79 65.46,38.03 65.66,38.23 95.38,38.23 97.54,40.39 102.23,40.39 104.65,42.8 104.65,44.96 105.41,45.72 JP8.8
P1.0  (via drill 0.25)
  Top 0.203: U1.20 43.49,23.17 JP17.2 | U7.46 26.74,37.92 27.05,38.23 27.05,38.61 26.29,39.37 26.29,40.13 v25.91,40.51
  Bottom 0.203: JP17.2 43.18,24.77 42.8,25.15 39.12,25.15 38.86,25.4 38.86,28.19 38.61,28.45 35.81,28.45 35.56,28.7 35.56,36.58 35.31,36.83 28.07,36.83 27.69,37.21 27.69,39.5 26.67,40.51 v25.91,40.51
P1.1  (via drill 0.25)
  Top 0.203: U1.21 44.26,22.67 44.07,22.48 44.07,21.72 43.94,21.59 JP17.4 | U7.47 26.34,38.43 25.53,39.24 v25.53,39.62 | v43.94,24.38 v41.91,24.38
  Bottom 0.203: v43.94,24.38 44.45,24.38 44.7,24.13 44.7,22.35 43.94,21.59 JP17.4 | v41.91,24.38 39.12,24.38 38.35,25.15 38.35,27.69 38.1,27.94 35.31,27.94 35.05,28.19 35.05,35.94 34.67,36.32 26.94,36.32 U7.47 26.34,39.32 26.04,39.62 v25.53,39.62
P1.2  (via drill 0.25)
  Top 0.203: U1.22 54.54,22.17 v54.61,22.1 | v95.25,11.3 95.25,13.21 95.5,13.46 99.19,13.46 99.57,13.08 102.74,13.08 103.12,13.46 S6.1
  Bottom 0.203: v54.61,22.1 53.85,22.1 52.07,20.32 52.07,14.61 52.45,14.22 57.4,14.22 58.04,13.59 58.04,9.27 58.42,8.89 95,8.89 95.25,9.14 v95.25,11.3
P1.3
  Top 0.203: U1.23 45.16,21.67 44.45,20.95 43.81,20.95 JP17.6
P1.4
  Top 0.203: U1.24 50.38,21.17 49.91,20.7 45.34,20.7 44.32,19.68 44.32,19.3 44.07,19.05 JP17.8
P3.0
  Top 0.203: U1.44 63.96,16.43 66.17,14.22 70.23,14.22 71.5,15.49 83.69,15.49 85.47,17.27 91.69,17.27 95.5,21.08 103,21.08 105.03,19.05 107.95,19.05 JP12.1
P3.1
  Top 0.203: U1.45 64.46,16.57 66.42,14.61 69.85,14.61 71.25,16 83.44,16 85.22,17.78 91.19,17.78 95.12,21.72 103.76,21.72 105.16,20.32 JP12.2
P3.2
  Top 0.203: U1.46 64.96,16.7 66.67,14.99 69.6,14.99 71.12,16.51 83.19,16.51 84.96,18.29 90.93,18.29 95,22.35 104.65,22.35 105.41,21.59 107.95,21.59 JP12.3
P3.3
  Top 0.203: U1.47 65.46,16.84 66.93,15.37 69.34,15.37 70.99,17.02 83.06,17.02 84.84,18.8 90.81,18.8 94.87,22.86 JP12.4
P3.4
  Top 0.203: U1.48 65.96,16.97 67.18,15.75 68.96,15.75 70.74,17.53 82.8,17.53 84.58,19.3 90.55,19.3 95.38,24.13 107.95,24.13 JP12.5
P3.5
  Top 0.203: U1.49 66.46,17.23 67.56,16.13 68.58,16.13 70.48,18.03 82.55,18.03 84.33,19.81 90.3,19.81 95.89,25.4 JP12.6
P3.6
  Top 0.203: U1.51 70.01,20.67 72.14,18.54 82.3,18.54 84.07,20.32 90.04,20.32 96.39,26.67 107.95,26.67 JP12.7
P3.7
  Top 0.203: U1.52 70.27,21.17 72.39,19.05 82.04,19.05 83.82,20.83 89.79,20.83 96.9,27.94 JP12.8
P4.0  (via drill 0.25)
  Top 0.203: U1.69 70.82,29.67 72.52,31.37 79.12,31.37 80.26,32.51 97.16,32.51 99.57,34.92 100.58,34.92 v101.6,35.94 | v101.6,41.15 JP9.2
  Route2 0.203: v101.6,35.94 v101.6,41.15
P4.1  (via drill 0.25)
  Top 0.203: U1.70 70.68,30.17 72.26,31.75 78.87,31.75 80.39,33.27 96.9,33.27 99.57,35.94 v100.33,35.94 | v100.33,41.15 100.33,49.53 JP9.1
  Route2 0.203: v100.33,35.94 v100.33,41.15
P4.2
  Top 0.203: U1.80 64.96,38.42 65.15,38.61 93.6,38.61 95.89,40.89 95.89,44.58 96.27,44.96 98.3,44.96 99.06,45.72 JP9.4
P4.3
  Top 0.203: U1.81 64.46,38.81 64.77,39.12 93.22,39.12 95.25,41.15 95.25,45.09 95.89,45.72 97.16,45.72 97.79,46.35 97.79,49.53 JP9.3
P4.4
  Top 0.203: U1.82 63.96,39.45 64.14,39.62 92.96,39.62 94.74,41.4 94.74,45.47 95.5,46.23 96.27,46.23 96.52,46.48 JP9.6
P4.5
  Top 0.203: U1.83 63.46,39.97 63.63,40.13 92.71,40.13 94.11,41.53 94.11,45.85 95.25,46.99 95.25,49.53 JP9.5
P4.6
  Top 0.203: U1.84 62.96,40.35 63.25,40.64 92.46,40.64 93.47,41.66 93.47,46.23 93.98,46.74 JP9.8
P4.7
  Top 0.203: U1.85 62.46,40.87 62.74,41.15 92.2,41.15 92.71,41.66 92.71,49.53 JP9.7
P5.0  (via drill 0.25)
  Top 0.203: U1.16 54.38,25.17 v54.86,25.65
  Bottom 0.203: v54.86,25.65 68.58,25.65 68.96,25.27 72.01,25.27 72.39,24.89 72.39,19.3 72.77,18.92 108.97,18.92 109.22,18.67 JP11.2
P5.1  (via drill 0.25)
  Top 0.203: U1.17 54.39,24.67 54.61,24.89 v55.5,24.89
  Bottom 0.203: v55.5,24.89 71.5,24.89 71.88,24.51 71.88,19.05 72.52,18.41 106.3,18.41 106.68,18.03 JP11.1
P5.2  (via drill 0.25)
  Top 0.203: U1.18 54.82,24.17 v54.86,24.13
  Bottom 0.203: v54.86,24.13 70.87,24.13 71.37,23.62 71.37,18.8 72.26,17.91 104.78,17.91 105.28,17.4 105.28,14.22 105.54,13.97 107.95,13.97 JP11.4
P5.3  (via drill 0.25)
  Top 0.203: U1.19 54.31,23.67 54.61,23.37 v55.5,23.37
  Bottom 0.203: v55.5,23.37 70.61,23.37 70.87,23.11 70.87,18.54 72.01,17.4 104.27,17.4 104.65,17.02 104.65,13.08 105.03,12.7 JP11.3
P5.4  (via drill 0.25)
  Top 0.203: U1.31 57.46,19.88 v56.64,20.7
  Bottom 0.203: v56.64,20.7 56.64,22.73 56.9,22.99 69.85,22.99 70.36,22.48 70.36,18.29 71.75,16.89 103.63,16.89 104.01,16.51 104.01,11.81 104.39,11.43 107.95,11.43 JP11.6
P5.5  (via drill 0.25)
  Top 0.203: U1.32 57.96,20.14 57.53,20.57 v57.53,21.21
  Bottom 0.203: v57.53,21.21 57.53,22.1 58.04,22.61 69.34,22.61 69.85,22.1 69.85,18.16 71.5,16.51 103.25,16.51 103.5,16.26 103.5,10.54 103.89,10.16 JP11.5
P5.6  (via drill 0.25)
  Top 0.203: U1.33 58.46,20.66 v58.42,20.7
  Bottom 0.203: v58.42,20.7 58.42,22.1 58.55,22.23 69.09,22.23 69.47,21.84 69.47,17.91 71.25,16.13 102.87,16.13 103.12,15.88 103.12,10.29 103.63,9.78 105.16,9.78 105.41,9.53 105.41,9.14 105.66,8.89 107.95,8.89 JP11.8
P5.7  (via drill 0.25)
  Top 0.203: U1.34 58.96,20.23 v59.44,20.7
  Bottom 0.203: v59.44,20.7 59.44,21.59 59.69,21.84 68.83,21.84 69.09,21.59 69.09,17.65 70.99,15.75 102.49,15.75 102.74,15.49 102.74,10.16 103.63,9.27 104.65,9.27 104.9,9.02 104.9,7.87 105.16,7.62 JP11.7
P12.0  (via drill 0.25)
  Top 0.203: U1.53 70.53,21.67 72.26,19.94 v73.41,19.94 | v75.18,14.73 77.34,14.73 78.87,13.21 78.87,8.38 79.38,7.87 90.3,7.87 91.44,6.73 JP10.3
  Route2 0.203: v73.41,19.94 73.41,16.51 v75.18,14.73
P12.1  (via drill 0.25)
  Top 0.203: U1.54 71.3,22.17 72.52,20.95 v74.42,20.95 | v79.12,14.73 79.12,14.61 80.26,13.46 80.26,9.91 81.03,9.14 93.22,9.14 93.98,8.38 JP10.4
  Route2 0.203: v74.42,20.95 74.42,16.76 76.45,14.73 v79.12,14.73
P12.2  (via drill 0.25)
  Top 0.203: U1.67 67.41,28.67 67.12,28.96 v67.06,28.96 | v81.79,13.34 81.79,10.79 82.68,9.91 95.89,9.91 96.52,9.27 JP10.5
  Route2 0.203: v67.06,28.96 67.06,26.04 67.31,25.78 76.2,25.78 76.71,26.29 80.52,26.29 80.9,25.91 80.9,14.1 81.66,13.34 v81.79,13.34
P12.3  (via drill 0.25)
  Top 0.203: U1.68 67.86,29.17 67.69,29.34 67.69,29.97 67.6,30.06 67.1,30.06 v67.06,30.1 | v81.79,14.48 82.8,14.48 83.19,14.1 83.19,11.3 83.82,10.67 94.23,10.67 94.36,10.54 97.03,10.54 99.06,8.51 JP10.6
  Route2 0.203: v67.06,30.1 68.07,30.1 68.45,29.72 72.26,29.72 72.64,29.34 72.64,27.3 73.28,26.67 81.03,26.67 81.41,26.29 81.41,14.86 v81.79,14.48
P12.6  (via drill 0.25)
  Top 0.203: U1.29 56.46,16.96 55.37,15.88 v55.37,15.62 | v97.92,11.43 101.22,11.43 101.6,11.05 JP10.7
  Bottom 0.203: v55.37,15.62 55.37,14.99 55.63,14.73 66.67,14.73 67.06,14.35 67.06,12.7 67.69,12.06 97.28,12.06 v97.92,11.43
P12.7  (via drill 0.25)
  Top 0.203: U1.30 56.96,16.7 56.52,16.26 v56.52,15.62 | v98.68,12.57 103.89,12.57 104.14,12.32 JP10.8
  Bottom 0.203: v56.52,15.62 67.18,15.62 67.69,15.11 67.69,12.95 68.07,12.57 v98.68,12.57
P15.0
  Top 0.203: U1.42 62.96,13.43 Y2.1 59.69,10.16 C14.1
P15.1
  Top 0.203: U1.43 63.46,14.01 Y2.2 67.31,10.16 C12.1
P15.2
  Top 0.203: U1.55 74.1,22.67 75.18,21.59 75.18,20.19 75.69,19.68 78.99,19.68 79.38,20.07 Y1.2 81.66,21.08 82.13,21.55 C18.1
P15.3
  Top 0.203: U1.56 71.94,23.17 72.9,24.13 C24.1 74.08,23.33 74.3,23.11 76.58,23.11 76.83,22.86 Y1.1
PSOC_D+_BUS  (via drill 0.25)
  Top 0.203: JP1.D+1 6.6,22.86 7.24,22.23 v7.62,22.23 | v54.23,13.34 R16.2
  Bottom 0.203: v7.62,22.23 8.51,22.23 9.27,22.99 20.83,22.99 22.1,21.72 24.51,21.72 25.65,20.57 27.43,20.57 28.83,19.18 28.83,12.83 29.72,11.94 51.94,11.94 52.32,11.56 52.83,11.56 53.34,12.06 53.34,13.21 53.47,13.34 v54.23,13.34
PSOC_D+_PAD
  Top 0.203: U1.35 59.46,17.55 58.93,17.02 58.17,17.02 57.66,16.51 57.66,13.84 57.15,13.34 R16.1
PSOC_D-_BUS  (via drill 0.25)
  Top 0.203: JP1.D-1 7.48,23.51 v7.62,23.37 | v52.58,12.32 54.1,12.32 54.36,12.06 R17.2
  Bottom 0.203: v7.62,23.37 21.08,23.37 22.35,22.1 24.77,22.1 25.91,20.95 27.69,20.95 29.21,19.43 29.21,13.08 29.97,12.32 v52.58,12.32
PSOC_D-_PAD
  Top 0.203: R17.1 57.78,12.06 58.42,12.7 58.42,16.13 58.8,16.51 59.56,16.51 59.96,16.91 U1.36
V_BUS_DEBUG  (via drill 0.25)
  Top 0.203: U7.18 32.41,29.82 v33.02,29.21 | v12.7,37.34 9.65,37.34 9.53,37.47 8.89,37.47
  Top 0.254: R5.2 8.89,37.47 R4.2
  Bottom 0.203: v33.02,29.21 30.48,31.75 23.88,31.75 23.75,31.62 22.35,31.62 21.59,32.38 21.59,37.47 21.21,37.85 16.89,37.85 16.38,37.34 v12.7,37.34
V_BUS_HOST  (via drill 0.25)
  Top 0.203: R3.2 13.58,28.79 | 13.58,28.79 R6.2 | 13.58,28.79 13.58,24.52 v13.97,24.13 | U1.27 55.46,16.98 54.1,15.62 52.32,15.62 52.07,15.88 52.07,18.54 51.82,18.8 v50.04,18.8
  Bottom 0.203: v13.97,24.13 17.78,24.13 18.03,23.88 22.35,23.88 22.86,23.37 26.42,23.37 26.67,23.62 30.23,23.62 30.48,23.37 30.48,18.92 31.62,17.78 39.75,17.78 40.01,17.53 40.01,16.51 40.39,16.13 46.61,16.13 47.37,15.37 49.02,15.37 49.53,15.88 49.53,18.29 v50.04,18.8
V_DEBUG
  Top 0.203: JP2.VBUS1 5.75,39.4
  Top 0.254: R4.1 8.89,41.91
  Top 0.508: 5.75,39.4 6.1,39.75 6.1,41.66 6.35,41.91 8.89,41.91 D2.A
V_HOST
  Top 0.203: JP1.VBUS1 5.87,24.16 6.35,24.64 | R3.1 12.7,26.04 12.95,25.78 12.95,24.89 12.7,24.64 D1.A
  Top 0.254: 11.18,24.64 D1.A
  Top 0.762: 6.35,24.64 11.18,24.64
V_IN  (via drill 0.51)
  Top 0.406: SJ1.2 18.8,19.05 | U2.1 21.4,17.46 21.08,17.78 | U2.3 21.4,15.56 | U3.1 21.4,25.08 21.08,25.4 | U3.3 21.4,23.18 21.08,22.86 | SJ2.2 16.38,46.23
  Top 0.762: 21.08,19.05 21.08,22.86 21.08,25.4 17.78,28.7 17.78,39.37 18.29,39.88 18.29,45.72 17.77,46.24 | 21.08,19.05 21.08,17.78 v21.08,15.88 21.4,15.56 | 18.8,19.05 21.08,19.05 | D4.C 17.77,46.24 | 17.77,46.24 17.76,46.23 16.38,46.23
  Bottom 1.016: JP6.1 66.04,3.81 65.53,4.32 45.34,4.32 42.29,1.27 16.51,1.27 15.24,2.54 15.24,14.35 16.13,15.24 20.44,15.24 v21.08,15.88
VCCA
  Top 0.203: U1.63 69.98,26.67 70.48,26.16 C1.1
VCCD  (via drill 0.25)
  Top 0.203: U1.86 61.96,33.29 v62.23,33.02 | 61.46,19.68 U1.39 61.46,17.41 61.98,16.89 61.98,15.49 61.85,15.37 61.79,15.31 C7.1
  Top 0.406: 61.46,19.68 61.46,20.31 61.47,20.32 v61.47,29.08
  Bottom 0.406: v62.23,33.02 62.23,29.84 v61.47,29.08
VDDIO  (via drill 0.25)
  Top 0.203: U1.50 66.96,17.5 67.56,16.89 v68.2,16.89 68.71,16.89 69.85,18.03 69.85,19.04 69.83,19.05 C9.1 | C15.1 70.23,34.67 70.36,34.54 70.36,33.66 | U1.75 70.14,32.67 70.36,32.89 70.36,33.66 | 70.36,33.66 v69.34,33.66 | U7.17 31.14,28.17 31.37,27.94 C27.1 32.06,28.9 v32,28.96 31.99,28.94 | U7.35 31.14,37.62 31.24,37.72 C29.1 32.19,38.68 v32.13,38.73 32.12,38.72 | U7.52 23.22,36.22 22.93,36.5 C31.1 23.37,37.59 v24,36.96 | U7.67 23.36,30.22 22.86,29.72 21.59,29.72 | 21.59,29.72 21.59,29.84 v21.21,30.23 | 21.59,29.72 21.59,29.21 | 21.59,29.21 21.59,28.97 | v54.61,20.32 54.96,19.97 U1.26 54.96,17.75 54.86,17.65 54.36,17.65 54.23,17.78 54.23,18.8 54.16,18.87 C13.1 | C25.1 21.64,29.16 21.59,29.21 | R8.2 R7.2 45.3,30.57 v45.21,30.48
  pour Route2 (isolate 0.305): 0,53.34 110.49,53.34 110.49,0 0,0
VDDIO_ARDUINO  (via drill 0.25, 0.51)
  Top 0.203: v55.24,33.02 54.96,33.3 U1.100 54.96,35.84 54.74,36.07 C11.1 | v80.64,31.75 85.09,31.75 JP13.2
  Top 1.016: S3.2 20.32,2.03 21.08,1.27 42.29,1.27 45.97,4.95 48.13,4.95 | 48.13,4.95 50.04,4.95 50.8,4.19 JP6.7 | 48.13,4.95 v48.13,6.86 | v48.13,10.03 v48.13,16.38
  Bottom 0.203: v55.24,33.02 59.44,33.02 60.58,34.16 62.99,34.16 64.14,33.02 64.14,32.26 64.64,31.75 v80.64,31.75
  Bottom 1.016: v48.13,6.86 v48.13,10.03 | v48.13,16.38 48.13,32.51 48.64,33.02 v55.24,33.02

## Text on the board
Top: 1
Route2: 2
Route15: 3
Bottom: 4 | v11
tPlace: GND | A4/SCL / P6.1 | A5/SDA / P6.0 | NC | GND | D13 / P6.7/SCK | D12/MISO / P6.6 | D11/MOSI / P6.5/PWM | D10/CS / P6.4/PWM | D9/PWM / P12.5 | D8 / P12.4 | D7 / P2.7 | D6/PWM / P2.6 | D5/PWM / P2.5 | D4 / P2.4 | D3/INT1 / P2.3/PWM | D2/INT0 / P2.2 | D1/TX / P2.1 | D0/RX / P2.0 | VDDIO | GND | 12.6 | 3.6 | 3.4 | 0.0 | VDDIO | 3.0 | 12.7 | 3.7 | 3.5 | 0.1 | 1.2 | 4.7 | 4.5 | 4.3 | 4.1 | 0.7 | 0.6 | GND | VDDIO | - | + | D BYPASS | DEBUGGER IO | 4.6 | 4.4 | 4.2 | 4.0 | 0.5 | 0.4 | I2C / ISO | USER LED / D13/P6.7 | 0.3 | 0.2 | DEBUGGER LED / P3.1 | DEBUGGER | 0.1 | 0.0 | SAR0 / BP | DelSig / BP | CY8C5888AXI-LP096 | GND | DEBUGGER BTN / P2.2 | SAR1 / BP | VDDIO | 3.7 | 3.6 | DEBUGGER / RESET | CY8C5868LTI-LP039 | 3.5 | 3.4 | TARGET | 3.3 | 3.2 | DEBUGGER / SWD PORT | USER BTN / P1.2 | 3.1 | 3.0 | TARGET / SWD PORT | TARGET / RESET | BATT / ISOLATE | 5.1 | 5.0 | V SEL | FreeSoC2 | 5.3 | 5.2 | VDDIO / 0 1 3 | PSoC5LP / Dev Board | 5.5 | 5.4 | 5.7 | 5.6 | ARDUINO / VDDIO2 | VDDIO | NC | VDDIO / ARDUINO | !RESET | 3.3V | 5V | GND | GND | V_IN | A0 / P15.5 | A1 / P15.4 | A2 / P6.3 | A3 / P6.2 | A4/SCL / P6.1 | A5/SDA / P6.0 | GND | VDDIO | SIO P12.0 | SIO P12.1 | SIO P12.2 | SIO P12.3 | SIO P12.6 | SIO P12.7 | GND | 2.5V-12V | 5V | 3.3V
Measures: Measurement units given in inches
tDocu: LAYER / NUMBERS | Mike Hord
